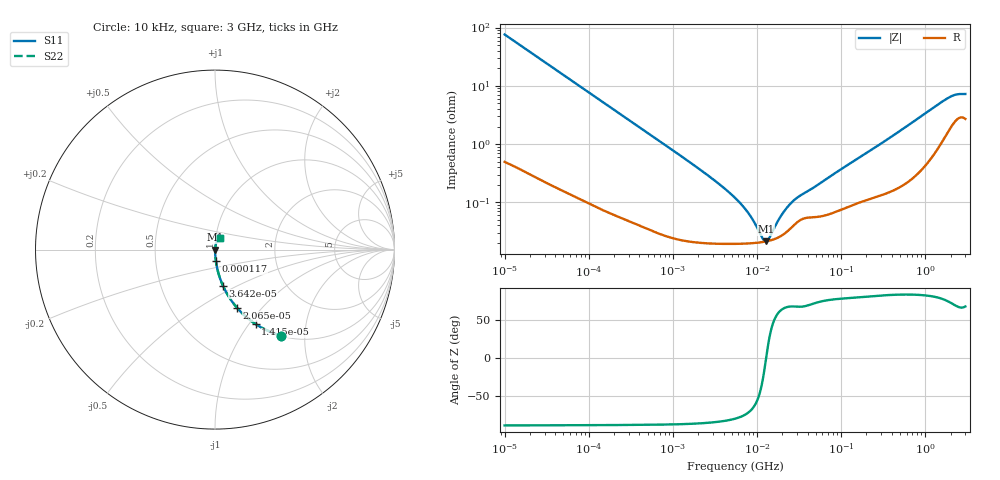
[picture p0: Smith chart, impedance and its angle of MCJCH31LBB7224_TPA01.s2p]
! MCJCH31LBB7224_TPA01  S-PARAMETER MODEL  ( Standard Model )
! Model Generated by TAIYO YUDEN Corporation (http://www.ty-top.com)
! Version 1.0
! TAIYO YUDEN Control No. 220601
! Copyright(c) 2015 TAIYO YUDEN CO.,LTD. All Rights Reserved.
! Product Description (link to TY-COMPAS)
! https://ds.yuden.co.jp/TYCOMPAS/or/detail?pn=MCJCH31LBB7224KTPA01&u=M
! Products Name : Multilayer Ceramic Capacitors
! Characteristics :
!  Capacitance : 0.22 [uF] , Rated Voltage : 100 [V] , TCC : X7R
!  Case Size : 3.2 x 1.6 / 0.126 x 0.063 [mm/inch] , Thickness : 1.6 / 0.063 [mm/inch]
!  (Conditions: Temperature = 25 [degC] , DC Bias Voltage = 0 [V])
! External Node Assignments :
!  1  o---| |---o  2
! GND o---------o GND
! Frequency Range : 10kHz  -  3GHz  [ 401 STEP ]
# MHZ S RI R 50
! Freq[MHz].  S11 Real  S11 Imag  S21 Real  S21 Imag  S12 Real  S12 Imag  S22 Real  S22 Imag
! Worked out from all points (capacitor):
!   401 points, 10 kHz to 3 GHz, reference 50 ohm
!   read as one part in series: C = 209 nF near 10.65 kHz
!   lowest |Z| = 21.3 mohm at 12.83 MHz (marker M1)
!   series resonance near 12.85 MHz, so ESL is about 740 pH
!   S11 on the Smith chart (normalised r, x): 10 kHz: 1.01, -1.52; 14.15 kHz: 1.01, -1.08; 20.65 kHz: 1.01, -0.74; 36.42 kHz: 1.00, -0.42; 117 kHz: 1.00, -0.13; 3 GHz: 1.05, +0.13
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0.01  0.3679 -0.479  0.6321 0.479  0.6321 0.479  0.3679 -0.479
0.014146  0.2269 -0.4152  0.7731 0.4152  0.7731 0.4152  0.2269 -0.4152
0.020651  0.1224 -0.3238  0.8776 0.3238  0.8776 0.3238  0.1224 -0.3238
0.036425  0.0441 -0.2007  0.9559 0.2007  0.9559 0.2007  0.0441 -0.2007
0.082683  0.00966 -0.0921  0.9903 0.0921  0.9903 0.0921  0.00966 -0.0921
0.11696  0.00518 -0.0656  0.9948 0.0656  0.9948 0.0656  0.00518 -0.0656
0.683653  0.000419 -0.0114  0.9996 0.0114  0.9996 0.0114  0.000419 -0.0114
2.737278  0.000204 -0.00274  0.9998 0.00274  0.9998 0.00274  0.000204 -0.00274
5.477226  0.000194 -0.00118  0.9998 0.00118  0.9998 0.00118  0.000194 -0.00118
7.747855  0.000197 -0.000649  0.9998 0.000649  0.9998 0.000649  0.000197 -0.000649
9.070798  0.000199 -0.000438  0.9998 0.000438  0.9998 0.000438  0.000199 -0.000438
11.67315  0.000208 -0.000119  0.9998 0.000119  0.9998 0.000119  0.000208 -0.000119
12.83117  0.000213 -1.5e-06  0.9998 1.5e-06  0.9998 1.5e-06  0.000213 -1.5e-06
14.10408  0.00022 0.000116  0.9998 -0.000116  0.9998 -0.000116  0.00022 0.000116
18.73182  0.000258 0.000482  0.9997 -0.000482  0.9997 -0.000482  0.000258 0.000482
24.10585  0.000338 0.000828  0.9997 -0.000828  0.9997 -0.000828  0.000338 0.000828
30.05882  0.000455 0.00111  0.9995 -0.00111  0.9995 -0.00111  0.000455 0.00111
45.28751  0.000554 0.00163  0.9994 -0.00163  0.9994 -0.00163  0.000554 0.00163
374.4521  0.00164 0.0125  0.9984 -0.0125  0.9984 -0.0125  0.00164 0.0125
1811.492  0.0181 0.0565  0.9819 -0.0565  0.9819 -0.0565  0.0181 0.0565
2331.196  0.029 0.0626  0.971 -0.0626  0.971 -0.0626  0.029 0.0626
3000  0.0304 0.0634  0.9696 -0.0634  0.9696 -0.0634  0.0304 0.0634
